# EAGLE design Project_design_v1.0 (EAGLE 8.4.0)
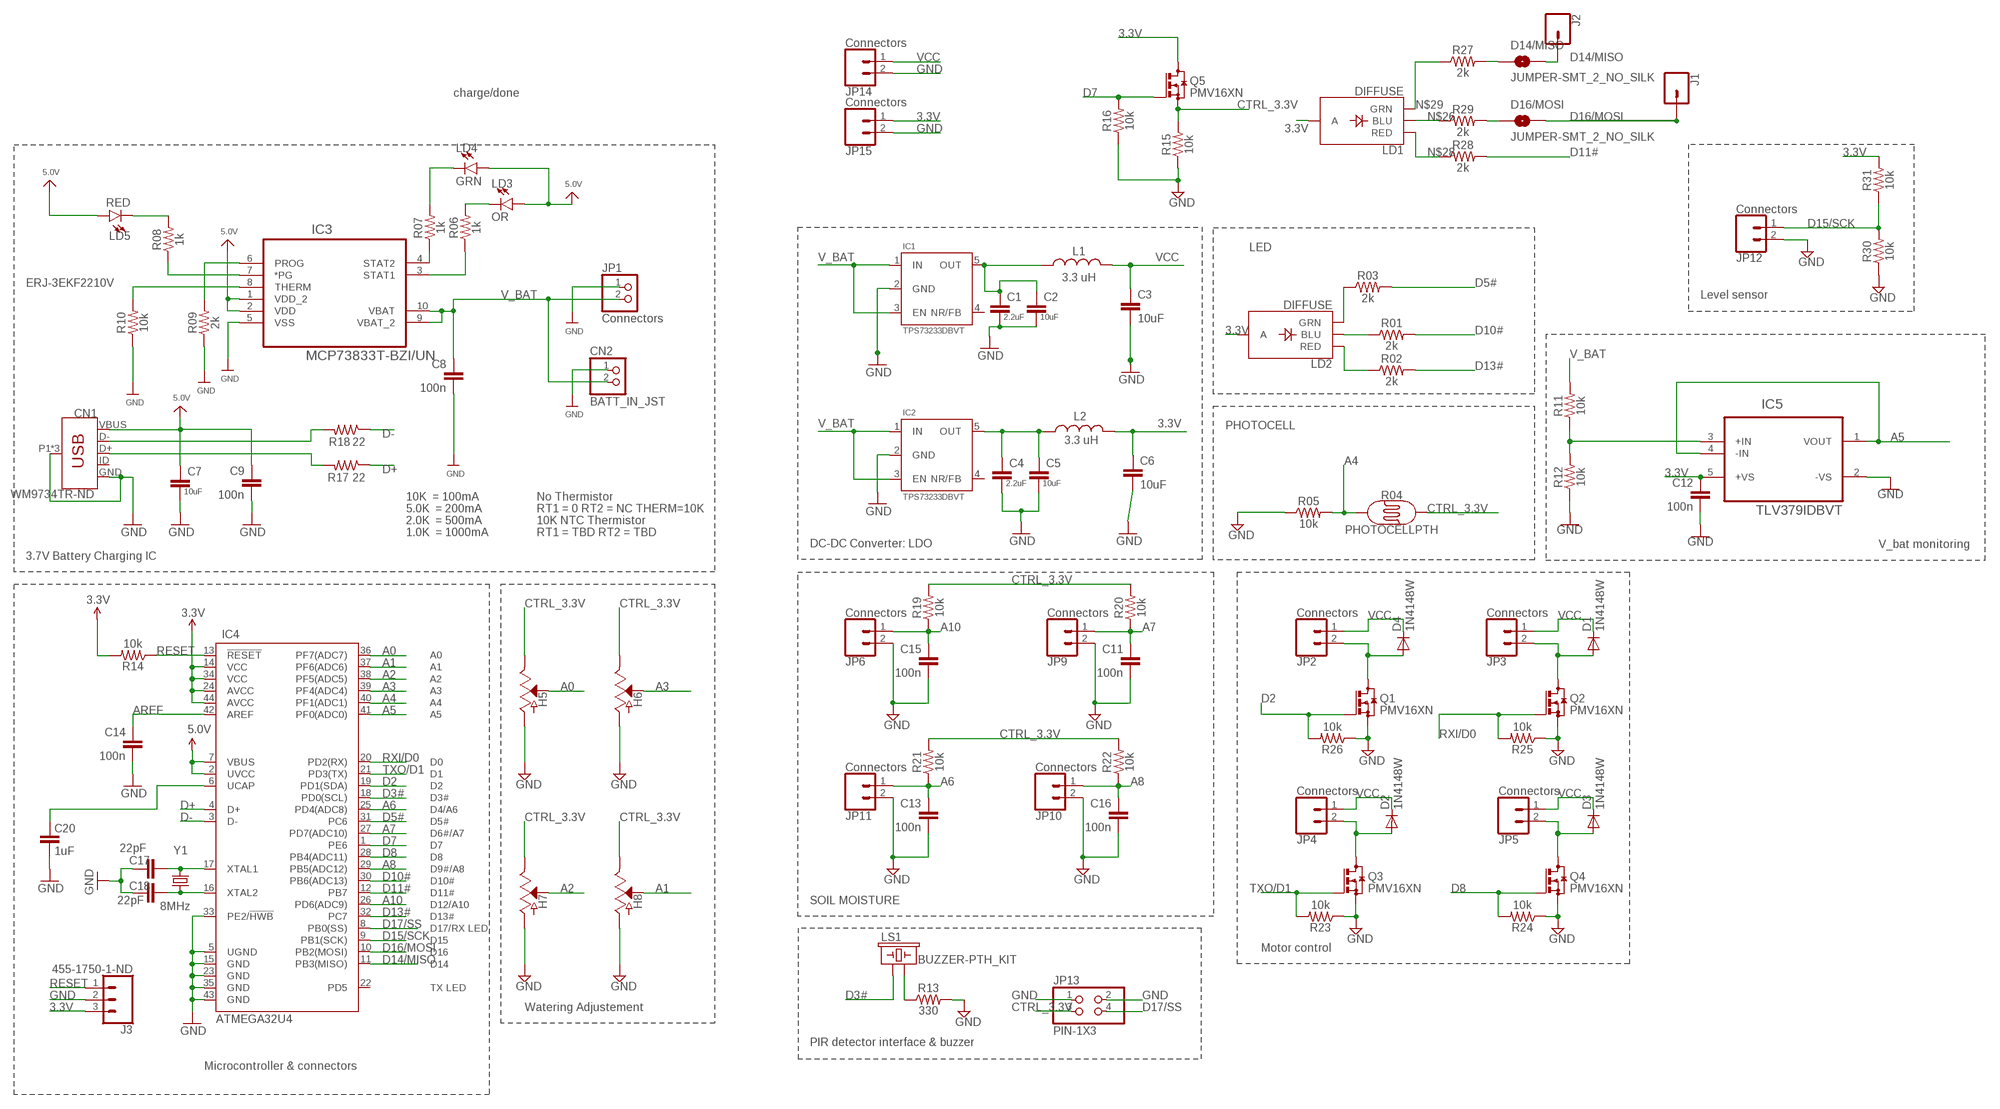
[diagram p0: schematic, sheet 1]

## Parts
C1  2.2uF  CAP0603-CAP  [0603-CAP]
C2  10uF  CAP0603-CAP  [0603-CAP]
C3  10uF  CAP0603-CAP  [0603-CAP]
C4  2.2uF  CAP0603-CAP  [0603-CAP]
C5  10uF  CAP0603-CAP  [0603-CAP]
C6  10uF  CAP0603-CAP  [0603-CAP]
C7  10uF  CAP0603-CAP  [0603-CAP]
C8  100n  CAPA0402  [0402]
C9  100n  CAPA0402  [0402]
C11  100n  CAPA0402  [0402]
C12  100n  CAPA0402  [0402]
C13  100n  CAPA0402  [0402]
C14  100n  CAPA0402  [0402]
C15  100n  CAPA0402  [0402]
C16  100n  CAPA0402  [0402]
C17  22pF  CAP0603-CAP  [0603-CAP]
C18  22pF  CAP0603-CAP  [0603-CAP]
C20  1uF  CAP0603-CAP  [0603-CAP]
CN1  WM9734TR-ND  USB_MICRO-B_FEMALE-SMT-VERT  [USB-B-MICRO-SMD_VERT]
CN2  BATT_IN_JST  JST_2PIN  [JSTPH2]
D1  1N4148W  CGRM4002-G  [SOD-123_MINI-SMA]
D2  1N4148W  CGRM4002-G  [SOD-123_MINI-SMA]
D3  1N4148W  CGRM4002-G  [SOD-123_MINI-SMA]
D4  1N4148W  CGRM4002-G  [SOD-123_MINI-SMA]
D14/MISO  JUMPER-SMT_2_NO_SILK  [SMT-JUMPER_2_NO_SILK]
D16/MOSI  JUMPER-SMT_2_NO_SILK  [SMT-JUMPER_2_NO_SILK]
H5  POT1  SOIL_MOISTURE  [SOIL_MOISTURE]
H6  POT2  SOIL_MOISTURE  [SOIL_MOISTURE]
H7  POT3  SOIL_MOISTURE  [SOIL_MOISTURE]
H8  POT4  SOIL_MOISTURE  [SOIL_MOISTURE]
IC1  TPS73233DBVT  TPS732XXDBV  [SOT23-5]
IC2  TPS73233DBVT  TPS732XXDBV  [SOT23-5]
IC3  MCP73833T-BZI/UN  [SOP50P490X110-10N]
IC4  ATMEGA32U4  ATMEGA32U4TQFP-44  [TQFP44]
IC5  TLV379IDBVT  AD8009JRTZ-REEL  [SOT95P280X145-5N]
J1  CONN_01  [1X01]
J2  CONN_01  [1X01]
J3  455-1750-1-ND  CONN_03  [1X03]
JP1  Connectors  PINHD-1X2  [1X02]
JP2  Connectors  CONN_02  [1X02]
JP3  Connectors  CONN_02  [1X02]
JP4  Connectors  CONN_02  [1X02]
JP5  Connectors  CONN_02  [1X02]
JP6  Connectors  CONN_02  [1X02]
JP9  Connectors  CONN_02  [1X02]
JP10  Connectors  CONN_02  [1X02]
JP11  Connectors  CONN_02  [1X02]
JP12  Connectors  CONN_02  [1X02]
JP13  PIN-1X3  PINHD-2X2  [2X02]
JP14  Connectors  CONN_02  [1X02]
JP15  Connectors  CONN_02  [1X02]
L1  3.3 uH  INDUCTOR0603  [0603]
L2  3.3 uH  INDUCTOR0603  [0603]
LD1  DIFFUSE  LED_RGB_THRU_CA  [LED-RGB_THRU_5MM]
LD2  DIFFUSE  LED_RGB_THRU_CA  [LED-RGB_THRU_5MM]
LD3  OR  LED3MM  [LED_3MM]
LD4  GRN  LED3MM  [LED_3MM]
LD5  RED  LED3MM  [LED_3MM]
LS1  BUZZER-PTH_KIT  [BUZZER-12MM-KIT]
Q1  PMV16XN  [SOT23]
Q2  PMV16XN  [SOT23]
Q3  PMV16XN  [SOT23]
Q4  PMV16XN  [SOT23]
Q5  PMV16XN  [SOT23]
R01  2k  0603RESIST  [0603]
R02  2k  0603RESIST  [0603]
R03  2k  0603RESIST  [0603]
R04  PHOTOCELLPTH  [PHOTOCELL]
R05  10k  0603RESIST  [0603]
R06  1k  0603RESIST  [0603]
R07  1k  0603RESIST  [0603]
R08  1k  0603RESIST  [0603]
R09  2k  0603RESIST  [0603]
R10  10k  0603RESIST  [0603]
R11  10k  0603RESIST  [0603]
R12  10k  0603RESIST  [0603]
R13  330  0603RESIST  [0603]
R14  10k  0603RESIST  [0603]
R15  10k  0603RESIST  [0603]
R16  10k  0603RESIST  [0603]
R17  22  RESISTOR0603-RES  [0603-RES]
R18  22  RESISTOR0603-RES  [0603-RES]
R19  10k  0603RESIST  [0603]
R20  10k  0603RESIST  [0603]
R21  10k  0603RESIST  [0603]
R22  10k  0603RESIST  [0603]
R23  10k  0603RESIST  [0603]
R24  10k  0603RESIST  [0603]
R25  10k  0603RESIST  [0603]
R26  10k  0603RESIST  [0603]
R27  2k  0603RESIST  [0603]
R28  2k  0603RESIST  [0603]
R29  2k  0603RESIST  [0603]
R30  10k  0603RESIST  [0603]
R31  10k  0603RESIST  [0603]
Y1  8MHz  CRYSTAL5X3  [CRYSTAL-SMD-5X3]

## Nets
3.3V: C6.1 C12.1 IC4.14(VCC) IC4.24(AVCC) IC4.34(VCC) IC4.44(AVCC) IC5.5(+VS) J3.3 JP15.1 L2.2 LD1.3(A) LD2.3(A) Q5.3(D) R14.2 R31.2
5.0V: C7.1 C9.1 CN1.VBUS IC3.1(VDD_2) IC3.2(VDD) IC4.2(UVCC) IC4.7(VBUS) LD3.A LD4.A LD5.A
A0: H5.3(VOUT) IC4.36(PF7(ADC7))
A1: H8.3(VOUT) IC4.37(PF6(ADC6))
A2: H7.3(VOUT) IC4.38(PF5(ADC5))
A3: H6.3(VOUT) IC4.39(PF4(ADC4))
A4: IC4.40(PF1(ADC1)) R04.1 R05.2
A5: IC4.41(PF0(ADC0)) IC5.1(VOUT) IC5.4(-IN)
A6: C13.1 IC4.25(PD4(ADC8)) JP11.1 R21.1
A7: C11.1 IC4.27(PD7(ADC10)) JP9.1 R20.1
A8: C16.1 IC4.29(PB5(ADC12)) JP10.1 R22.1
A10: C15.1 IC4.26(PD6(ADC9)) JP6.1 R19.1
AREF: C14.1 IC4.42(AREF)
CTRL_3.3V: H5.1(VCC) H6.1(VCC) H7.1(VCC) H8.1(VCC) JP13.3 Q5.2(S) R04.2 R15.2 R19.2 R20.2 R21.2 R22.2
D2: IC4.19(PD1(SDA)) Q1.1(G) R26.2
D3#: IC4.18(PD0(SCL)) LS1.+
D5#: IC4.31(PC6) R03.2
D7: IC4.1(PE6) Q5.1(G) R16.2
D8: IC4.28(PB4(ADC11)) Q4.1(G) R24.2
D10#: IC4.30(PB6(ADC13)) R01.2
D11#: IC4.12(PB7) R28.2
D13#: IC4.32(PC7) R02.2
D14/MISO: D14/MISO.2 IC4.11(PB3(MISO)) J2.1
D15/SCK: IC4.9(PB1(SCK)) JP12.1 R30.2 R31.1
D16/MOSI: D16/MOSI.2 IC4.10(PB2(MOSI)) J1.1
D17/SS: IC4.8(PB0(SS)) JP13.4
D+: IC4.4(D+) R17.1
D-: IC4.3(D-) R18.1
GND: C1.2 C2.2 C3.2 C4.2 C5.2 C6.2 C7.2 C8.2 C9.2 C11.2 C12.2 C13.2 C14.2 C15.2 C16.2 C17.2 C18.2 C20.1 CN1.GND CN1.P1(SHIELD) CN1.P2(SHIELD) CN1.P3(SHIELD) CN2.1 H5.2(GND) H6.2(GND) H7.2(GND) H8.2(GND) IC1.2(GND) IC2.2(GND) IC3.5(VSS) IC4.5(UGND) IC4.15(GND) IC4.23(GND) IC4.33(PE2/!HWB) IC4.35(GND) IC4.43(GND) IC5.2(-VS) J3.2 JP1.1 JP6.2 JP9.2 JP10.2 JP11.2 JP12.2 JP13.1 JP13.2 JP14.2 JP15.2 Q1.2(S) Q2.2(S) Q3.2(S) Q4.2(S) R05.1 R09.1 R10.1 R12.1 R13.2 R15.1 R16.1 R23.1 R24.1 R25.1 R26.1 R30.1
N$1: LD2.2(GRN) R03.1
N$2: C4.1 C5.1 IC2.5(OUT) L2.1
N$3: LD3.K(C) R06.2
N$4: LD4.K(C) R07.2
N$5: IC3.4(STAT2) R07.1
N$6: IC3.3(STAT1) R06.1
N$7: IC3.7(*PG) R08.1
N$8: IC3.8(THERM) R10.2
N$9: C18.1 IC4.16(XTAL2) Y1.1
N$10: D4.A JP2.2 Q1.3(D)
N$11: D1.A JP3.2 Q2.3(D)
N$12: LD5.K(C) R08.2
N$13: C1.1 C2.1 IC1.5(OUT) L1.1
N$14: D2.A JP4.2 Q3.3(D)
N$15: D3.A JP5.2 Q4.3(D)
N$16: IC3.6(PROG) R09.2
N$17: IC5.3(+IN) R11.1 R12.2
N$18: C17.1 IC4.17(XTAL1) Y1.3
N$19: C20.2 IC4.6(UCAP)
N$20: CN1.D- R18.2
N$21: CN1.D+ R17.2
N$22: LS1.- R13.1
N$26: LD1.1(BLU) R29.1
N$28: LD1.4(RED) R28.1
N$29: LD1.2(GRN) R27.1
N$30: D16/MOSI.1 R29.2
N$32: D14/MISO.1 R27.2
N$34: LD2.1(BLU) R01.1
N$35: LD2.4(RED) R02.1
RESET: IC4.13(!RESET) J3.1 R14.1
RXI/D0: IC4.20(PD2(RX)) Q2.1(G) R25.2
TXO/D1: IC4.21(PD3(TX)) Q3.1(G) R23.2
V_BAT: C8.1 CN2.2 IC1.1(IN) IC1.3(EN) IC2.1(IN) IC2.3(EN) IC3.9(VBAT_2) IC3.10(VBAT) JP1.2 R11.2
VCC: C3.1 D1.C D2.C D3.C D4.C JP2.1 JP3.1 JP4.1 JP5.1 JP14.1 L1.2
Unconnected: CN1.ID IC1.4(NR/FB) IC2.4(NR/FB) IC4.22(PD5)

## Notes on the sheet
- charge/done
- LED
- ERJ-3EKF2210V
- Level sensor
- PHOTOCELL
- 10K  = 100mA | No Thermistor
- 5.0K  = 200mA | RT1 = 0 RT2 = NC THERM=10K
- 2.0K  = 500mA | 10K NTC Thermistor
- 1.0K  = 1000mA | RT1 = TBD RT2 = TBD
- DC-DC Converter: LDO | V_bat monitoring
- 3.7V Battery Charging IC
- SOIL MOISTURE
- Motor control
- Watering Adjustement
- PIR detector interface & buzzer
- Microcontroller & connectors

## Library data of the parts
C1 C4 = SparkFun-Passives:CAP: Capacitor; PARTNO: C1608X7S1C225K080AC
C2 C3 C5-C7 = SparkFun-Passives:CAP: Capacitor; PARTNO: GRM188R60J106ME47D
C8 C9 C11-C16 = custom_part:CAPA; PARTNO: CGA2B3X7R1E104K050BB
C17 C18 = SparkFun:CAP: Capacitor; PARTNO: CL10C2R2BB8NNNC
C20 = SparkFun:CAP: Capacitor; PARTNO: CL10B105KP8NNNC
CN1 = SparkFun-Connectors:USB_MICRO-B: USB Type Micro-B Connector Male/female and PTH/SMT variants SparkFun Products: SparkFun microB USB Breakout SparkFun USB microB Plug Breakout SparkFun ESP8266 Thing; PARTNO: 1051330011; PROD_ID: CONN-13534
CN2 = microbuilder:JST_2PIN: JST 2-Pin Right-Angle Connector; PARTNO: B2B-XH-A(LF)(SN)
D1-D4 = diode:CGRM400*-G: Molded plasitc,JEDEC SOD-123/Mini SMA; PARTNO: 1N4148W
D14/MISO D16/MOSI = SparkFun-Jumpers:JUMPER-SMT_2_NO: Normally open jumper
H5-H8 = potentiometer:SOIL_MOISTURE; PARTNO: SEN-13322
IC1 IC2 = TPS32xx:TPS732XX: Cap-Free, NMOS, 250mA Low Dropout Regulator with Reverse Current Protection; PARTNO: TPS73233DBVT
IC3 = MCP73833T-BZI_UN:MCP73833T-BZI/UN: LI-ION/LI-POLY CONTROLLERS; AVAILABILITY: Good; DESCRIPTION: Linear Charge Management Controller Li-Ion/Li-Pol 1mA 4.2V/4.35V/4.4V/4.5V 10-Pin MSOP T/R; MF: Microchip; MP: MCP73833T-BZI/UN; PACKAGE: MSOP-10 Microchip; PRICE: 0.72 USD
IC4 = ATMEGA32U4:ATMEGA32U4: Atmel 44-pin 8-bit Microcontroller with 32KBytes of ISP Flash and USB Controller; AVAILABILITY: Good; DESCRIPTION: Embedded microcontroller ATMEGA32U4RC-AU TQFP 44 (10x10) Microchip Technology 8-Bit 16 MHz I/O number 26; MF: Microchip; MP: ATMEGA32U4RC-AU; PACKAGE: TQFP-44 Microchip; PARTNO: ATMEGA32U4RC-MUR; PRICE: 3.89 USD
IC5 = AD8009JRTZ-REEL:AD8009JRTZ-REEL: Low Distortion Amplifier; AVAILABILITY: Unavailable; DESCRIPTION: Ic Opamp Cfa 845mhz Sot23-5; MF: Analog Devices; MP: AD8009JRTZ-REEL; PACKAGE: SOT-23-5 Analog Devices; PARTNO: TLV379IDBVT; PRICE: 1.92 USD
J1 J2 = SparkFun-Connectors:CONN_01: Single connection point. Often used as Generic Header-pin footprint for 0.1 inch spaced/style header connections
J3 = SparkFun-Connectors:CONN_03: Multi connection point. Often used as Generic Header-pin footprint for 0.1 inch spaced/style header connections On any of the 0.1 inch spaced packages, you can populate with these: Break Away Headers - Straight (PRT-00116) Break Away Male Headers - Right Angle (PRT-00553) Female Headers (PRT-00115)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; PROD_ID: XXX-00000
JP1 = pinhead:PINHD-1X2: PIN HEADER; PARTNO: /
JP2-JP6 JP9-JP12 JP14 JP15 = SparkFun-Connectors:CONN_02: Multi connection point. Often used as Generic Header-pin footprint for 0.1 inch spaced/style header connections; PARTNO: M20-9960245
JP13 = pinhead:PINHD-2X2: PIN HEADER; PARTNO: M22-2040805
L1 L2 = SparkFun-Passives:INDUCTOR: Inductors; PARTNO: LQM18PN3R3MGHD
LD1 LD2 = RGB_LED:LED_RGB_THRU_CA; PARTNO: WP154A4SEJ3VBDZGW/CA
LD3 = SparkFun-LED:LED: LED (Generic); PARTNO: TLHO4600; PROD_ID: DIO-08794
LD4 = SparkFun-LED:LED: LED (Generic); PARTNO: TLLG4400; PROD_ID: DIO-08794
LD5 = SparkFun-LED:LED: LED (Generic); PARTNO: TLHK4600; PROD_ID: DIO-08794
LS1 = SparkFun-Electromechanical:BUZZER: Buzzer; PARTNO: CEM-1203(42); PROD_ID: COMP-08253; SF_SKU: COM-07950
Q1-Q5 = custom_part_2:PMV16XN; PARTNO: PMV16XNR
R01-R03 R09 R27-R29 = custom_part:0603RESIST; PARTNO: ERJ-PA3F2001V
R04 = SparkFun-Sensors:PHOTOCELL: Photocell (Photodetector, Photo Resistor, CdS); PARTNO: 1528-2141-ND; PROD_ID: COMP-09129; SF_ID: SEN-09088
R05 R10-R12 R14-R16 R19-R26 R30 R31 = custom_part:0603RESIST; PARTNO: ERA-3AEB103V
R06-R08 R13 = custom_part:0603RESIST; PARTNO: RC0603JR-07330RL
R17 R18 = SparkFun:RESISTOR: Resistor; PARTNO: RC0603JR-0722RL
Y1 = SparkFun:CRYSTAL: Crystals; PARTNO: ABM3C-8.000MHZ-D4Y-T

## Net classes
7 GND: width 0.152 mm, clearance 0.2 mm

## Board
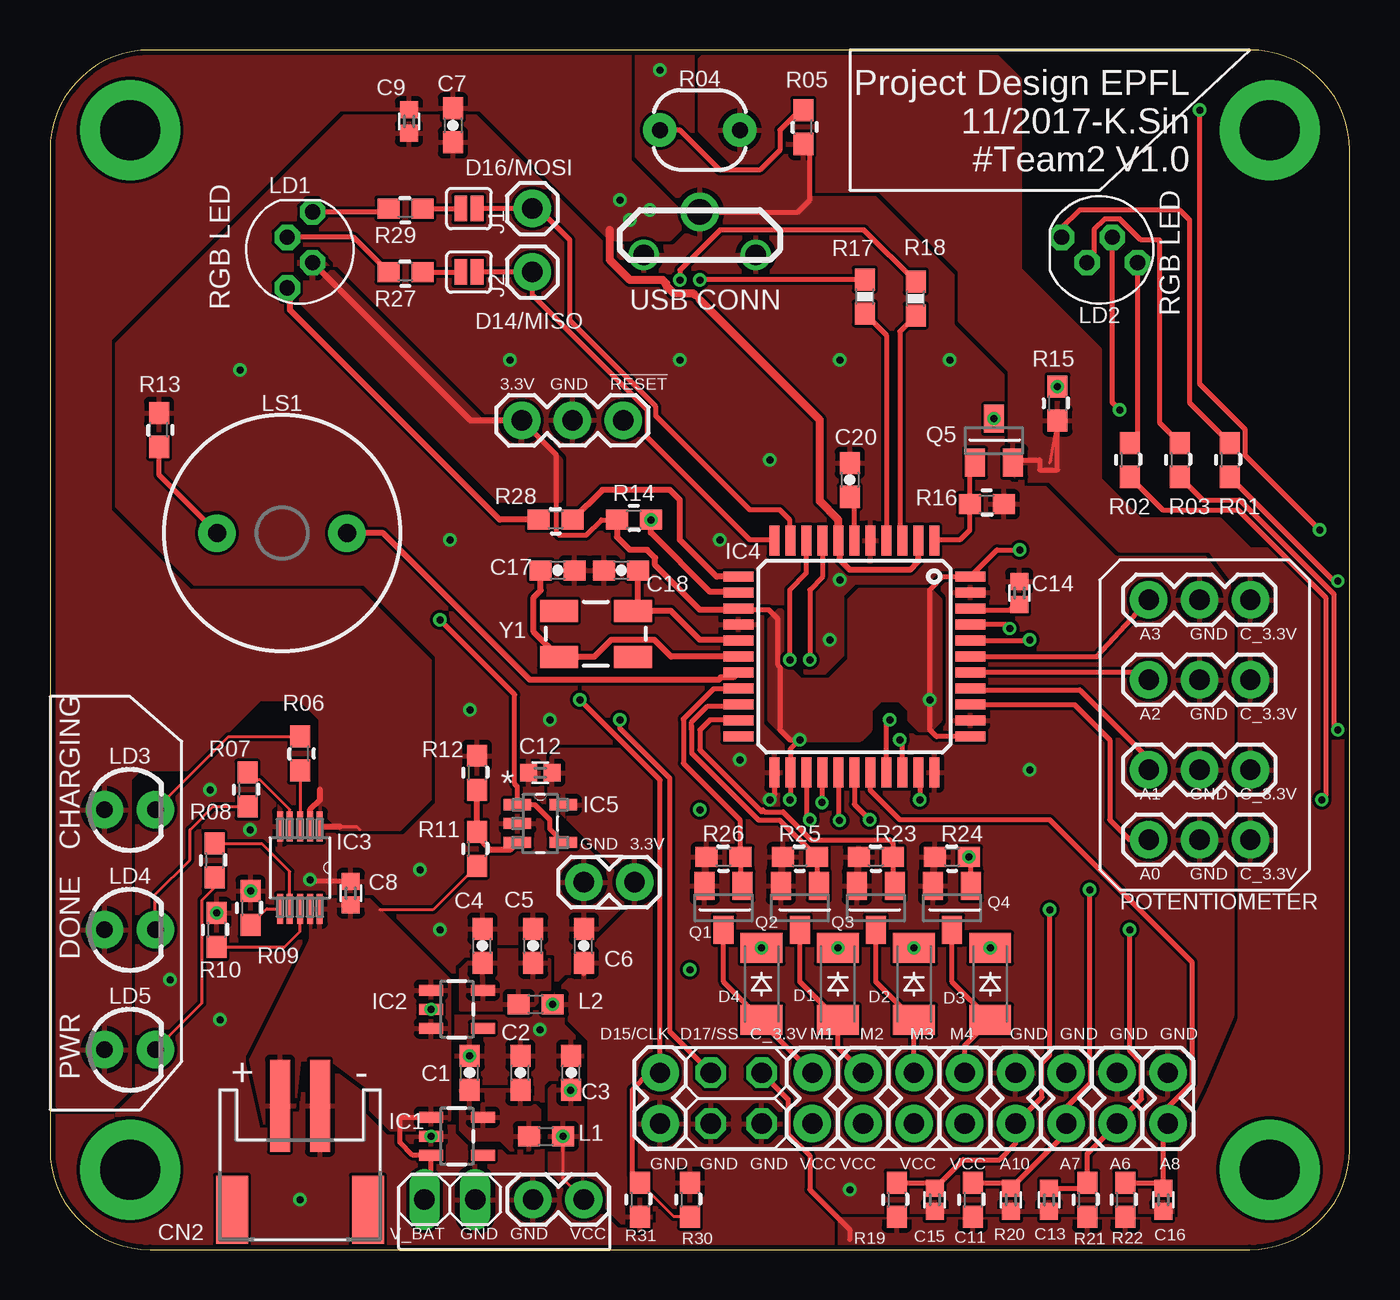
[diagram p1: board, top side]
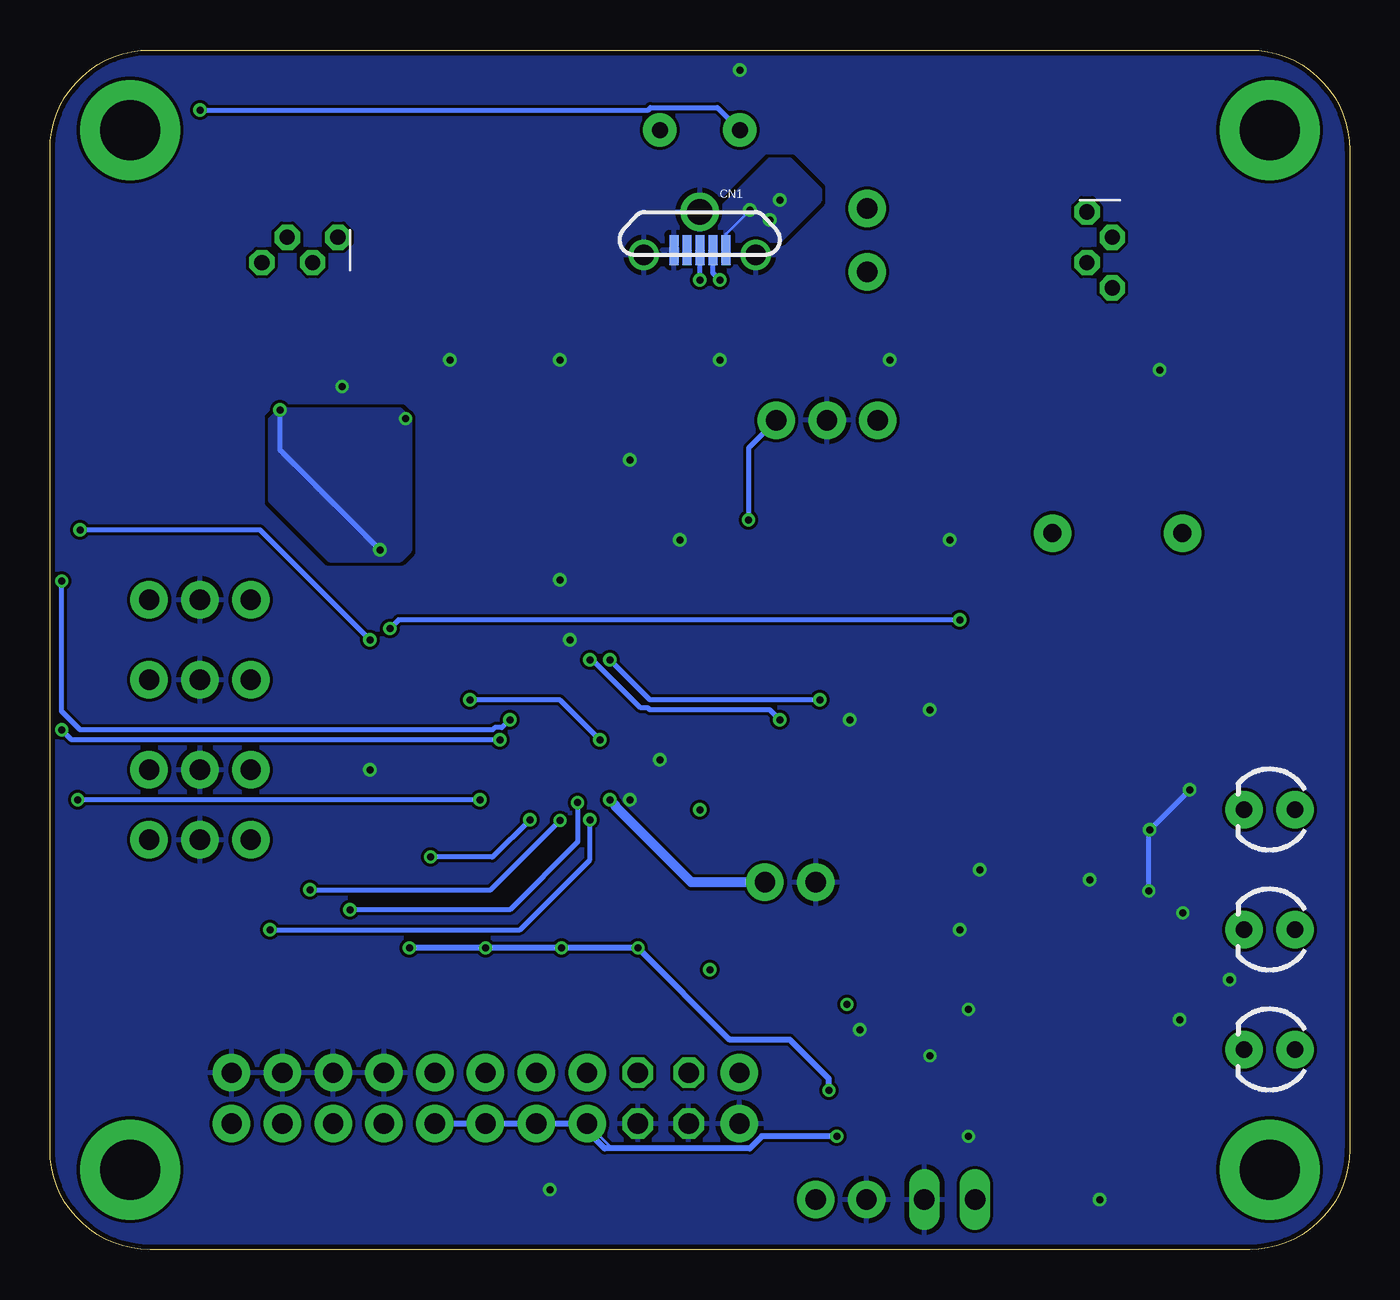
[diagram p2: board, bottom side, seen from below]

Size 65 x 60 mm. Coordinates in mm from the lower left corner, seen from the top.
Outline: 0,55 0,5 arc90 5,0 60,0 arc90 65,5 65,55 arc90 60,60 5,60 arc90 0,55
Copper layers (1*16): Top 0.035mm / dielectric 1.5mm / Bottom 0.035mm
Design rules "SeeedStudio_2layer_DRU_no_angle_20140221": minimum track width 6mil, minimum drill 12mil, track to track 6mil, track to pad 6mil, pad to pad 6mil, via to via 6mil, smd to smd 0mil, copper to edge 10mil, drill to drill 10mil, minimum pad ring 10mil, minimum via ring 6mil, stop-mask expansion 2mil, vias tented up to drill 100mil, thermal gap 10mil

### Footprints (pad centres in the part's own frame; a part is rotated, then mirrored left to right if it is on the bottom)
0603-CAP = smd 1.1 x 1: 1 -0.85,0; 2 0.85,0
0402 = smd 0.85 x 0.9: 1 -0.58,0; 2 0.58,0
USB-B-MICRO-SMD_VERT = smd 0.45 x 1.5: D+ 0,0; D- -0.65,0; GND 1.3,0; ID 0.65,0; VBUS -1.3,0 | drill 1.016: P1 -2.8,0.25; P2 2.8,0.25 | drill 1.27: P3 0,-1.9
JSTPH2 = smd 1 x 4.6: 1 -1,-3.7; 2 1,-3.7 | smd 1.6 x 3.4: NC1 -3.4,1.5; NC2 3.4,1.5
SOD-123_MINI-SMA = smd 1.5 x 2.1: A 1.8,0; C -1.8,0
SMT-JUMPER_2_NO_SILK = smd 0.635 x 1.27: 1 -0.406,0; 2 0.406,0
SOIL_MOISTURE = drill 1.016 pad 1.88: 1 -2.54,0; 2 0,0; 3 2.54,0
SOT23-5 = smd 0.55 x 1.2: 1 -0.95,-1.3; 2 0,-1.3; 3 0.95,-1.3; 4 0.95,1.3; 5 -0.95,1.3
SOP50P490X110-10N = smd 1.499 x 0.305: 1 -2.057,0.991; 2 -2.057,0.508; 3 -2.057,0; 4 -2.057,-0.508; 5 -2.057,-0.991; 6 2.057,-0.991; 7 2.057,-0.508; 8 2.057,0; 9 2.057,0.508; 10 2.057,0.991
TQFP44 = smd 1.5 x 0.5: 1 -5.8,4; 2 -5.8,3.2; 3 -5.8,2.4; 4 -5.8,1.6; 5 -5.8,0.8; 6 -5.8,0; 7 -5.8,-0.8; 8 -5.8,-1.6; 9 -5.8,-2.4; 10 -5.8,-3.2; 11 -5.8,-4; 23 5.8,-4; 24 5.8,-3.2; 25 5.8,-2.4; 26 5.8,-1.6; 27 5.8,-0.8; 28 5.8,0; 29 5.8,0.8; 30 5.8,1.6; 31 5.8,2.4; 32 5.8,3.2; 33 5.8,4 | smd 0.5 x 1.5: 12 -4,-5.8; 13 -3.2,-5.8; 14 -2.4,-5.8; 15 -1.6,-5.8; 16 -0.8,-5.8; 17 0,-5.8; 18 0.8,-5.8; 19 1.6,-5.8; 20 2.4,-5.8; 21 3.2,-5.8; 22 4,-5.8; 34 4,5.8; 35 3.2,5.8; 36 2.4,5.8; 37 1.6,5.8; 38 0.8,5.8; 39 0,5.8; 40 -0.8,5.8; 41 -1.6,5.8; 42 -2.4,5.8; 43 -3.2,5.8; 44 -4,5.8
SOT95P280X145-5N = smd 1.372 x 0.559: 1 -1.143,0.94; 2 -1.143,0; 3 -1.143,-0.94; 4 1.143,-0.94; 5 1.143,0.94
1X01 = drill 1.016 pad 1.88: 1 0,0
1X03 = drill 1.016 pad 1.88: 1 0,0; 2 2.54,0; 3 5.08,0
1X02 = drill 1.016 long: 1 -1.27,0; 2 1.27,0
1X02' = drill 1.016 pad 1.88: 1 0,0; 2 2.54,0
2X02 = drill 1.016 octagon: 1 -1.27,-1.27; 2 -1.27,1.27; 3 1.27,-1.27; 4 1.27,1.27
0603 = smd 1.1 x 1: 1 -0.85,0; 2 0.85,0
LED-RGB_THRU_5MM = drill 0.762 pad 1.27 octagon: 1 1.905,-0.635; 2 0.635,0.635; 4 -1.905,0.635 | drill 0.75 pad 1.27 octagon: 3 -0.635,-0.635
LED_3MM = drill 0.813 pad 1.88: A -1.27,0; K 1.27,0
BUZZER-12MM-KIT = drill 0.9 pad 1.88: + 3.25,0; - -3.25,0
SOT23 = smd 1 x 1.4: 1 -0.95,-1.1; 2 0.95,-1.1; 3 0,1.1
PHOTOCELL = drill 0.8 pad 1.676: 1 -2,0; 2 2,0
0603-RES = smd 1.1 x 1: 1 -0.85,0; 2 0.85,0
CRYSTAL-SMD-5X3 = smd 1.9 x 1.1: 1 -1.85,-1.15; 2 1.85,-1.15; 3 1.85,1.15; 4 -1.85,1.15

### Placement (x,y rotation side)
C1  20.99,8.84 90 top
C2  23.53,8.84 90 top
C3  26.07,8.84 90 top
C4  21.62,15.19 90 top
C5  24.16,15.19 90 top
C6  26.7,15.19 90 top
C7  20.16,56.23 270 top
C8  15.04,17.82 90 top
C9  17.96,56.43 270 top
C11  48.06,2.49 270 top
C12  24.52,23.85 180 top
C13  49.97,2.49 270 top
C14  48.48,32.84 90 top
C15  44.26,2.49 270 top
C16  55.69,2.49 270 top
C17  25.39,33.97 0 top
C18  28.57,33.97 180 top
C20  40,38.5 270 top
CN1  32.5,50 180 bottom
CN2  12.5,3.5 180 top
D1  39.41,13.29 270 top
D2  43.22,13.29 270 top
D3  47.02,13.29 270 top
D4  35.59,13.29 270 top
D14/MISO  20.95,48.9 0 top
D16/MOSI  20.95,52.07 0 top
H5  57.5,20.5 180 top
H6  57.5,32.5 180 top
H7  57.5,28.5 180 top
H8  57.5,24 180 top
IC1  20.36,5.67 270 top
IC2  20.36,12.02 270 top
IC3  12.51,19.09 270 top
IC4  40.23,29.66 270 top
IC5  24.52,21.31 0 top
J1  24.13,52.07 90 top
J2  24.13,48.9 90 top
J3  28.68,41.48 180 top
JP1  20,2.5 180 top
JP2  Connectors  [1X02']  38.13,6.3 90 top
JP3  Connectors  [1X02']  40.67,6.3 90 top
JP4  Connectors  [1X02']  43.22,6.3 90 top
JP5  Connectors  [1X02']  45.76,6.3 90 top
JP6  Connectors  [1X02']  48.3,6.3 90 top
JP9  Connectors  [1X02']  50.84,6.3 90 top
JP10  Connectors  [1X02']  55.91,6.3 90 top
JP11  Connectors  [1X02']  53.38,6.3 90 top
JP12  Connectors  [1X02']  30.52,8.84 270 top
JP13  34.33,7.57 90 top
JP14  Connectors  [1X02']  26.7,2.5 180 top
JP15  Connectors  [1X02']  29.24,18.38 180 top
L1  24.8,5.67 0 top
L2  24.29,12.27 0 top
LD1  12.5,50 90 top
LD2  52.5,50 180 top
LD3  4,22 0 top
LD4  4,16 0 top
LD5  4,10 0 top
LS1  11.61,35.84 0 top
Q1  33.69,17.09 180 top
Q2  37.5,17.09 180 top
Q3  41.31,17.09 180 top
Q4  45.12,17.09 180 top
Q5  47.22,40.45 0 top
R01  59,39.5 270 top
R02  54,39.5 270 top
R03  56.5,39.5 270 top
R04  32.5,56 0 top
R05  37.67,56.15 90 top
R06  12.51,24.81 90 top
R07  9.88,23 270 top
R08  8.23,19.46 270 top
R09  10.04,17.09 270 top
R10  8.33,15.98 270 top
R11  21.35,20.04 270 top
R12  21.35,23.85 270 top
R13  5.45,41 90 top
R14  29.2,36.51 180 top
R15  50.39,42.32 270 top
R16  46.85,37.28 180 top
R17  40.76,47.66 90 top
R18  43.3,47.56 90 top
R19  42.35,2.49 270 top
R20  46.16,2.49 270 top
R21  51.88,2.49 270 top
R22  53.78,2.49 270 top
R23  41.31,19.64 0 top
R24  45.12,19.64 0 top
R25  37.5,19.64 0 top
R26  33.69,19.64 0 top
R27  17.78,48.9 0 top
R28  25.3,36.51 0 top
R29  17.78,52.07 0 top
R30  32,2.5 270 top
R31  29.5,2.5 270 top
Y1  27.3,30.8 180 top

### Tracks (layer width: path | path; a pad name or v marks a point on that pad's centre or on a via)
3.3V  (via drill 0.35)
  Top 0.254: J3.3 25.32,39.76 25.32,35.89 25.48,35.73 26.81,35.73 27.58,36.5 R14.2 | v53.5,42 53.13,42.37 LD2.3 | v48.5,35 47.37,35 IC4.44 44.66,33.66 44,33 v44,27.5 44,26 44.34,25.66 IC4.34 | v37,22.5 37.03,22.53 IC4.24 37.03,25.03 v37.5,25.5 37,25.5 36.5,26 36.5,29.14 36.39,29.25 36.39,31.55 35.94,32 34.49,32 IC4.14
  Top 0.305: 26.7,13.83 C6.1 | IC4.14 34.37,32 32.5,32 30.27,34.23 30.27,34.6 29.87,35 29,35 28.36,35.65 R14.2 | LD1.3 21.02,41.48 J3.3
  Bottom 0.254: v37.5,25.5 39.5,27.5 v44,27.5 | v48.5,35 53.5,40 v53.5,42
  Bottom 0.508: v37,22.5 36.73,22.23 36.73,22.2 32.91,18.38 JP15.1
  other vias: 25.14,12.27 47.22,41.55
  pour Top (rank 2): 29,2.5 30,2.5 30,1 29,1 27,3 27,10 27,10.5 25.5,12 25,12 25,12.5 26.5,14 26.5,14.5 29,17 29,18 28.5,18.5 28.5,19 27,20.5 26.5,21 25.5,22 25,22.5 25,24.5 25.5,25 28.5,25 30,23.5 30,10
  pour Bottom: 47,41.5 47.5,42 53.5,42 54,41.5 54,37.5 51,34.5 47.5,34.5 47,35
  pour Top: 37.5,25.5 37,25.5 36,26.5 36,31.5 36.5,32 37,31.5 37,29 37.5,28.5 38,28.5 39,28.5 40,29.5 40,32.5 40.5,33 43.5,33 44,33 44.5,32.5 44.5,27.5 44.5,26.5 44,26 43.5,26 43,26.5 43,27 42.5,27.5 41.5,27.5 41,27 41,26.5 41,26 40.5,25.5
  pour Top (rank 2): 25.5,37.5 22.5,37.5 12.5,47.5 12.5,49.5 13.5,49.5 21.5,41.5 22,41.5 23.5,41.5 25.5,39.5
5.0V  (via drill 0.35)
  Top 0.152: 14.5,21.15 15.35,21.15 15.5,21 | 13.5,22.5 13.01,22.01 | v30,52 29.5,52 v29,51.5
  Top 0.254: 43.43,35 IC4.2 | 39.5,35 39.5,35.39 IC4.7
  Top 0.305: 43.43,35 43.43,34.43 43,34 40,34 39.5,34.5 39.5,35 | 32.5,47.5 32.25,47.75 | IC3.1 14.5,21.15 | IC3.2 13.01,22.01 13.5,22.5 13.5,23
  Top 0.406: IC4.7 39.43,36.5 38.5,37.43 38.5,41.5 32.5,47.5 | 32.25,47.75 32.18,47.82 31.22,47.82 30.82,48.22 30.82,48.32 30.64,48.5 29,48.5 28,49.5 28,51
  Bottom 0.152: CN1.VBUS 31.2,50.8 v30,52
  other vias: 28.5,52.5
  pour Top: 4,23.5 4,8 3,7 0.5,7 -0.5,8 -0.5,60 0.5,61 22.5,61 27.5,61.5 29,61.5 29,54.5 31.5,52 31.5,51 31,50.5 28,50.5 21.5,57 14.5,57 3,45.5 3,37 7,33 15.5,33 19,29.5 19,22.5 17.5,21 14.5,21 13.5,22 13.5,26.5 12.5,27.5 10.5,27.5 7,24 4.5,24
  pour Bottom: 31,50.5 28.5,50.5 26.5,52.5 26.5,53 28,54.5 29,54.5 31.5,52 31.5,51
A0
  Top 0.254: IC4.36 51.24,27.26 53,25.5 53,21.5 54,20.5 H5.3
A1
  Top 0.254: IC4.37 46.09,28 51.5,28 54.96,24.54 H8.3
A2
  Top 0.254: H7.3 54.63,28.86 IC4.38
A3
  Top 0.254: IC4.39 52.37,29.66 H6.3
A4  (via drill 0.35)
  Top 0.254: IC4.40 48.96,30.46 v49,30.5 | v63.5,36 59.78,39.72 59.78,41.02 57.5,43.3 v57.5,57 | R05.2 37.5,57 36.5,56 36.5,55 35.5,54 33.5,54 31.5,56 R04.1
  Bottom 0.254: v49,30.5 54.5,36 v63.5,36 | v57.5,57 35.08,57 34.96,57.12 31.62,57.12 R04.1
A5  (via drill 0.35)
  Top 0.254: v19.5,31.5 23.24,27.76 23.24,23.28 23.38,23.14 IC5.1 24.25,22.25 25,21.5 25,21.04 IC5.4 | v48,31.07 47.81,31.26 IC4.41
  Bottom 0.254: v19.5,31.5 47.57,31.5 v48,31.07
A6  (via drill 0.35)
  Top 0.254: C13.1 51.6,3.07 R21.1 51.88,4.8 JP11.1 54.59,7.52 54.59,9.35 54,9.94 v54,16 | IC4.25 37.83,21.67 v38,21.5
  Bottom 0.254: v54,16 41.5,16 38,19.5 v38,21.5
A7  (via drill 0.35)
  Top 0.254: R20.1 47.8,3.34 C11.1 50.84,5.84 JP9.1 50.84,7.12 52.05,8.34 52.05,9.35 52,9.4 v52,18 | IC4.27 39.43,21.53 v39.5,21.46
  Bottom 0.254: v52,18 42.96,18 v39.5,21.46
A8
  Top 0.254: R22.1 55.66,3.34 56,3 55.76,3 C16.1 55.69,6.07 JP10.1 55.91,7.12 57.13,8.34 57.13,14.37 50,21.5 42.5,21.5 41.03,22.97 IC4.29
A10  (via drill 0.35)
  Top 0.254: R19.1 43.98,3.34 C15.1 45.69,4.5 47.5,4.5 48.3,5.29 JP6.1 49.62,7.62 49.62,9.35 50,9.73 v50,17 | IC4.26 38.61,23.84 v38.61,22.35
  Bottom 0.254: v38.61,22.35 38.61,21 | 38.61,21 38.61,20.89 | 38.61,21 38.61,20.39 42,17 v50,17
AREF
  Top 0.254: IC4.42 46.09,32 48,32 48.26,32.26 C14.1
CTRL_3.3V
  Top 0.152: R15.2 50.01,39.35
  Top 0.254: JP13.3 36.92,7.52 36.92,5.79 38,4.71 38,3 40,1 40,0.5 | Q5.2 48.16,39.5 49.5,39.5 49.5,39 50.39,39 R15.2
  pour Top: 39.5,1.5 39.5,-1.5 40,-2 64,-2 68,2 68,33 67,34 62.5,34 61.5,35 60,35 58.5,36.5 54.5,36.5 52.5,38.5 52.5,45 48.5,49 48.5,58.5 45.5,61.5 34.5,61.5 32.5,59.5 32.5,56 34.5,54 36,54 37,53 41.5,53 45.5,49 45.5,46.5 48,44 48,39 48.5,38.5 50,38.5 53.5,35 58,35 59.5,33 59.5,11.5 58,8 56.5,5 56.5,1.5
D2
  Top 0.254: Q1.1 34.54,18.3 R26.2 34.5,19.68 34.5,21.5 31.69,24.31 31.69,26.5 | 31.69,26.55 31.69,26.5 | 31.69,26.5 31.69,26.55 | 31.69,26.55 33.2,28.06 IC4.19
D3#
  Top 0.305: IC4.18 34.19,28.61 33.55,28.61 33.44,28.5 24,28.5 16.66,35.84 LS1.+
D5#  (via drill 0.35)
  Top 0.254: R03.2 57.65,37.5 59.5,37.5 64.21,32.79 64.21,26.2 v64.41,26 | IC4.31 42.63,25.37 v42.5,25.5
  Bottom 0.254: v42.5,25.5 63.91,25.5 v64.41,26
D7
  Top 0.254: IC4.1 44.27,35.5 45.5,35.5 46,36 R16.2 46,39.09 Q5.1
D8  (via drill 0.35)
  Top 0.254: IC4.28 40.23,22.27 v41,21.5 | R24.2 46.05,19.55 46.05,18.21 Q4.1
  Bottom 0.254: v41,21.5 42.87,19.64 R24.2
  other vias: 45.97,19.64
D10#  (via drill 0.35)
  Top 0.254: IC4.30 41.83,26.33 v42,26.5 | R01.2 64.21,33.44 v64.42,33.44
  Bottom 0.254: v42,26.5 42.39,26.11 42.75,26.11 42.86,26 63.5,26 64.42,26.92 v64.42,33.44
D11#
  Top 0.305: IC4.12 33.34,33.66 33,34 31.5,35.5 31.5,37.5 31,38 27.64,38 R28.2
D13#  (via drill 0.35)
  Top 0.254: R02.2 55.65,37 59.42,37 63.81,32.62 63.81,22.7 v63.61,22.5 | IC4.32 43.5,23.79 v43.5,22.5
  Bottom 0.254: v43.5,22.5 v63.61,22.5
D14/MISO
  Top 0.254: D14/MISO.2 J2.1 24.13,47.75 29.89,41.98 29.89,40.61 35,35.5 36.19,35.5 IC4.11
D15/SCK  (via drill 0.35)
  Top 0.152: R30.2 31.2,1.65 R31.1
  Top 0.254: R31.1 29.13,3.72 29.13,8 29.97,8.84 JP12.1 30.52,23.48 v26.5,27.5 | v37,29.5 37,33 37.83,33.83 IC4.9
  Bottom 0.254: v26.5,27.5 35,27.5 v37,29.5
D16/MOSI
  Top 0.254: D16/MOSI.2 J1.1 24.43,52.07 26,50.5 26,46.45 30.3,42.15 30.3,41.7 35,37 36.5,37 37,36.5 37,35.49 IC4.10
D17/SS  (via drill 0.35)
  Top 0.254: JP13.4 31,10.89 31,23.57 28.5,26.07 v28.5,26.5 | v38,29.5 38,33 38.63,33.63 IC4.8
  Bottom 0.254: v28.5,26.5 29,27 35,27 35.09,27.09 35.45,27.09 37.86,29.5 v38,29.5
D+
  Top 0.254: R17.1 41.83,45.74 IC4.4
D-
  Top 0.254: R18.1 42.5,45.91 42.5,35.59 IC4.3
GND  (via drill 0.35)
  Top 0.254: CN1.P3 37.4,51.9 38,52.5 38,54.98 R05.1 | IC4.23 36.23,22.73 v36,22.5 | C8.2 13.1,18.41 v13,18.5
  Bottom 0.254: v10.04,17.93 10.04,20.96 v10,21 v8,23
  other vias: 50.39,43.17 19.05,12.02 20.99,9.69 19.05,5.67 8.33,16.84 23,44.5 31.5,44.5 39.5,44.5 45,44.5 9.5,44 6,13.5 8.5,11.5 40,3 49,24 12.5,2.5 20,35.5 21,27 19.5,16 39,30.5 36,39.5 30.5,59 24.5,11 33.5,35.5 39.5,33.5 34.5,24.5 18.5,19 25,26.5
  pour Top (rank 6): -6,-4 -6,64 71,64 71,-4
  pour Bottom (rank 6): -5,-4.5 -5,64 70.5,64 71,-5.5 -4.5,-5.5
N$1
  Top 0.254: R03.1 55.5,41.35 55.5,50.5 54.56,50.5 53.51,51.55 52.76,51.55 52.22,51.01 52.22,49.72 LD2.2
N$2
  pour Top: 20.5,12 24,12 25,13 25,14.5 24.5,15 21.5,15 20.5,14
N$3
  Top 0.152: LD3.K 8.93,25.66 R06.2
N$4
  Top 0.152: LD4.K 5.27,17.77 7,19.5 7,21 8.15,22.16 R07.2
N$5
  Top 0.152: IC3.4 12,22 10.5,23.5 10,23.5 9.88,23.62 R07.1
N$6
  Top 0.152: R06.1 IC3.3
N$7
  Top 0.152: IC3.7 12,18.9 10.6,20.3 R08.1
N$8
  Top 0.152: R10.2 11.73,15.13 12.51,15.9 IC3.8
N$9
  Top 0.305: IC4.16 34.39,30.5 32.5,30.5 31.05,31.95 Y1.1 29.42,32.22 C18.1
N$10
  Top 0.254: JP2.2 35.59,11.38 D4.A 33.69,13.39 Q1.3
N$11
  Top 0.254: JP3.2 39.41,10.11 D1.A 37.5,13.39 Q2.3
N$12
  Top 0.152: R08.2 8.23,18.11 7.6,17.48 7.6,12.33 LD5.K
N$13
  pour Top: 20.5,8 20.5,6 21,5.5 22.5,5.5 23,5 24,5 24.5,5.5 24.5,7 24,7.5 24,8
N$14
  Top 0.254: JP4.2 D2.A 41.31,13.39 Q3.3
N$15
  Top 0.254: JP5.2 45.76,10.21 D3.A 45.12,13.39 Q4.3
N$16
  Top 0.152: R09.2 10.84,17.04 IC3.6
N$17
  Top 0.305: IC5.3 23.01,20 22.02,20 21.35,20.67 R11.1 R12.2
N$18
  Top 0.305: IC4.17 31.07,29.66 30.23,30.5 28.07,30.5 27.22,29.64 Y1.3 24.2,30.9 24.2,32.62 24.55,32.97 C17.1
N$19
  Top 0.254: IC4.6 40.23,37.92 C20.2
N$20  (via drill 0.35)
  Top 0.254: R18.2 40.72,51 33.5,51 31.5,49 v31.5,48.5
  Bottom 0.254: v31.5,48.5 31.85,48.85 CN1.D-
N$21  (via drill 0.35)
  Top 0.254: R17.2 32.52,48.52 v32.5,48.5
  Bottom 0.254: v32.5,48.5 CN1.D+
N$22
  Top 0.254: LS1.- 5.45,38.74 R13.1
N$23  (via drill 3 pad 5)
  other vias: 4,56
N$24  (via drill 3 pad 5)
  other vias: 61,56
N$25  (via drill 3 pad 5)
  other vias: 61,4
N$26
  Top 0.254: LD1.1 16.77,51.91 R29.1
N$27  (via drill 3 pad 5)
  other vias: 4,4
N$28
  Top 0.305: R28.1 22.49,36.51 12,47 12,47.96 LD1.4
N$29
  Top 0.254: R27.1 15.19,50.63 LD1.2
N$30
  Top 0.254: R29.2 D16/MOSI.1
N$32
  Top 0.254: R27.2 D14/MISO.1
N$34
  Top 0.254: R01.1 57,42.35 57,51.5 56.5,52 51.5,52 50.59,51.09 LD2.1
N$35
  Top 0.254: R02.1 54.41,40.76 LD2.4
N$36  (via drill 0.35)
  other vias: 32,14
N$37  (via drill 0.35)
  other vias: 32.5,22
RESET  (via drill 0.35)
  Top 0.305: IC4.13 34.4,32.89 33.02,32.89 30.05,35.86 v30.05,36.5 R14.1
  Bottom 0.254: J3.1 30.05,40.1 v30.05,36.5
RXI/D0
  Top 0.254: Q2.1 38.35,18.3 R25.2 36.5,21.49 35.44,21.49 32.09,24.83 32.09,26 | 32.09,26.17 32.09,26 | 32.09,26 32.09,26.38 32.89,27.18 34.35,27.18 IC4.20
TXO/D1
  Top 0.254: Q3.1 42.16,18.3 42.16,19.5 | 42.16,19.5 R23.2 | IC4.21 34.39,26.5 33,26.5 32.5,26 32.5,25 35.5,22 | 35.5,22 35.61,21.89 | 35.5,22 35.64,22 35.75,21.89 36.67,21.89 38.06,20.5 42,20.5 42.16,20.34 42.16,19.5
V_BAT
  Top 0.152: R11.2 19.16,17 16.5,17
  Top 0.254: JP1.2 19.05,2.5 IC1.3 18.14,4.71 17.5,5.36 17.5,6.5 17.61,6.62 IC1.1
  pour Top: 12,5 12.5,9.5 14,9.5 16,8 16,7 17,6 19.5,6 20,6.5 20,13.5 16,17.5 13,17.5 13,15.5 10,9.5 11,5
VCC  (via drill 0.35)
  Top 0.152: JP14.1 25.65,3.55 L1.2 | C3.1 v26.04,7.96 25.65,7.57
  Bottom 0.152: L1.2 29.5,5.67 30.03,5.13 36.97,5.13 JP2.1 38.5,6.3 JP3.1 41,6.3 JP4.1 43.5,6.3 45.5,6.3 JP5.1
  Bottom 0.254: 43.13,15 D2.C
  Bottom 0.305: L1.2 29.39,5.67 30,5.05 37.26,5.05 38.5,6.3 | JP2.1 41,6.3 | JP3.1 43.5,6.3 | JP4.1 45.5,6.3 | v26.04,7.96 26.04,8.54 28,10.5 31.01,10.5 D4.C D1.C 43.05,15.09 43.13,15 | D2.C D3.C
  other vias: 25.65,5.67 35.59,15.09 39.41,15.09 43.22,15.09 47.02,15.09
  pour Top (rank 3): 27,2.5 27,8 26.5,8.5 26,8.5 25.5,8.5 25,8 25,4 26,3 26,2.5

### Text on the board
tPlace: Project Design EPFL / 11/2017-K.Sin / #Team2 V1.0 | RGB LED | RGB LED | USB CONN | 3.3V | GND | !RESET | A3 | GND | C_3.3V | A2 | GND | C_3.3V | A1 | GND | C_3.3V | CHARGING | GND | 3.3V | A0 | GND | C_3.3V | POTENTIOMETER | DONE | D15/CLK | D17/SS | C_3.3V | M1 | M2 | M3 | M4 | GND | GND | GND | GND | PWR | GND | GND | GND | VCC | VCC | VCC | VCC | A10 | A7 | A6 | A8 | V_BAT | GND | GND | VCC
Mechanical: LED RGB 5mm diam / LED R/G/O 3mm diam

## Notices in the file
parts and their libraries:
SparkFun-Sensors: Licensing: Creative Commons ShareAlike 4.0 International - https://creativecommons.org/licenses/by-sa/4.0
SparkFun-Passives: Licensing: CC v3.0 Share-Alike You are welcome to use this library for commercial purposes.
